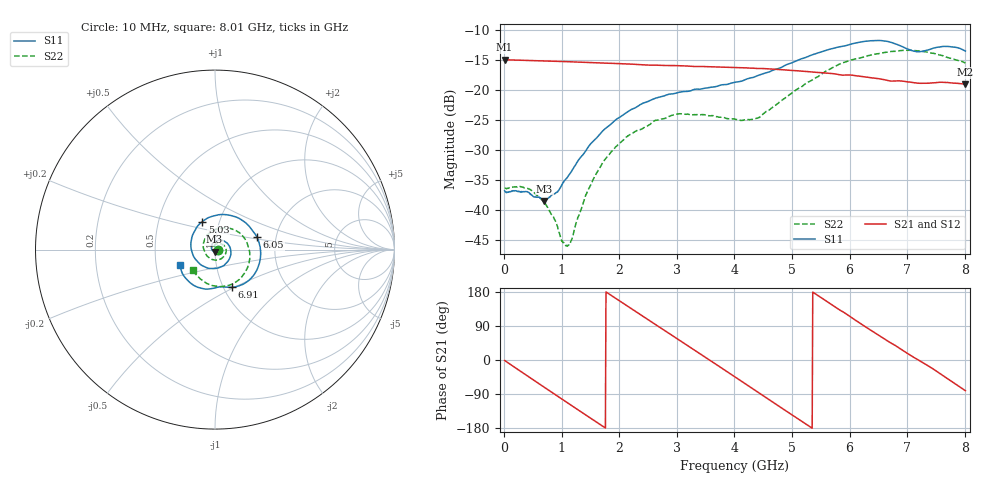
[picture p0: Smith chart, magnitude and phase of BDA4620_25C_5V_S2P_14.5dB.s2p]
!Agilent Technologies,E5071B,MY42404982,A.09.10
!Date: Wed May 06 09:01:15 2026
!Data & Calibration Information:
!Freq	S11:SOLT2(ON)	S21:SOLT2(ON)	S12:SOLT2(ON)	S22:SOLT2(ON)
# Hz S RI R 50
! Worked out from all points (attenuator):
!   801 points, 10 MHz to 8.01 GHz, reference 50 ohm
!   highest |S21| = -14.92 dB at 10 MHz (marker M1); lowest = -19.1 dB at 8.01 GHz (marker M2)
!   lowest |S11| = -38.5 dB at 700 MHz (marker M3), VSWR 1.02, Z = 49.8 - j1.16 ohm
!   |S11| at or under -10 dB: start of sweep to end of sweep
!   |S22| runs from -46.1 to -13.3 dB; largest |S21 - S12| = 0.00077
!   S11 on the Smith chart (normalised r, x): 10 MHz: 1.03, -0.00; 5.03 GHz: 0.83, +0.27; 6.05 GHz: 1.59, +0.23; 6.91 GHz: 1.10, -0.49; 8.01 GHz: 0.67, -0.12
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1e7  0.0144 -0.00103  0.1794 -0.00382  0.1797 -0.00389  0.0151 -0.000625
4.3e8  0.00882 -0.0108  0.1261 -0.1237  0.1261 -0.124  0.0134 -0.00665
7e8  -0.00204 -0.0117  0.054 -0.1667  0.0539 -0.1669  0.00734 -0.00885
9.2e8  -0.0123 -0.00687  -0.0136 -0.1732  -0.0137 -0.1734  0.000829 -0.00734
1.09e9  -0.0184 0.00155  -0.0641 -0.1604  -0.0642 -0.1606  -0.00418 -0.00285
1.17e9  -0.0196 0.00704  -0.0857 -0.1491  -0.0861 -0.1494  -0.0056 -0.000168
1.35e9  -0.02 0.0199  -0.1273 -0.1139  -0.1274 -0.1141  -0.00753 0.00725
1.58e9  -0.0117 0.0368  -0.1602 -0.0541  -0.1605 -0.0541  -0.00573 0.0183
1.9e9  0.015 0.0523  -0.1622 0.0391  -0.1624 0.0392  0.00645 0.0313
2.68e9  0.0869 0.00214  0.00416 0.1611  0.00443 0.1614  0.0533 0.0179
3.4e9  0.0351 -0.0954  0.1506 0.0452  0.1509 0.0451  0.0455 -0.0424
4.01e9  -0.0826 -0.0815  0.1098 -0.1087  0.1099 -0.1089  -0.0217 -0.053
4.42e9  -0.1329 0.00373  0.0106 -0.1511  0.0104 -0.1513  -0.0581 -0.00998
5.03e9  -0.0699 0.1565  -0.1231 -0.0777  -0.1234 -0.0777  -0.0316 0.0912
5.35e9  0.0272 0.195  -0.1414 -0.000164  -0.1416 -0.000186  0.0289 0.1176
6.05e9  0.2338 0.069  -0.046 0.1248  -0.0459 0.125  0.1723 0.0503
6.37e9  0.25 -0.0638  0.0259 0.1241  0.026 0.1243  0.194 -0.0279
6.68e9  0.1784 -0.1798  0.0798 0.0892  0.0801 0.0895  0.177 -0.1098
6.91e9  0.0953 -0.2105  0.1063 0.0533  0.1066 0.0534  0.1406 -0.1617
7.19e9  0.0268 -0.2071  0.114 0.00056  0.1143 0.000551  0.0675 -0.2019
7.57e9  -0.082 -0.2141  0.0943 -0.068  0.0945 -0.0679  -0.0364 -0.1924
8.01e9  -0.1943 -0.0838  0.0175 -0.1101  0.0177 -0.1104  -0.1215 -0.1164
